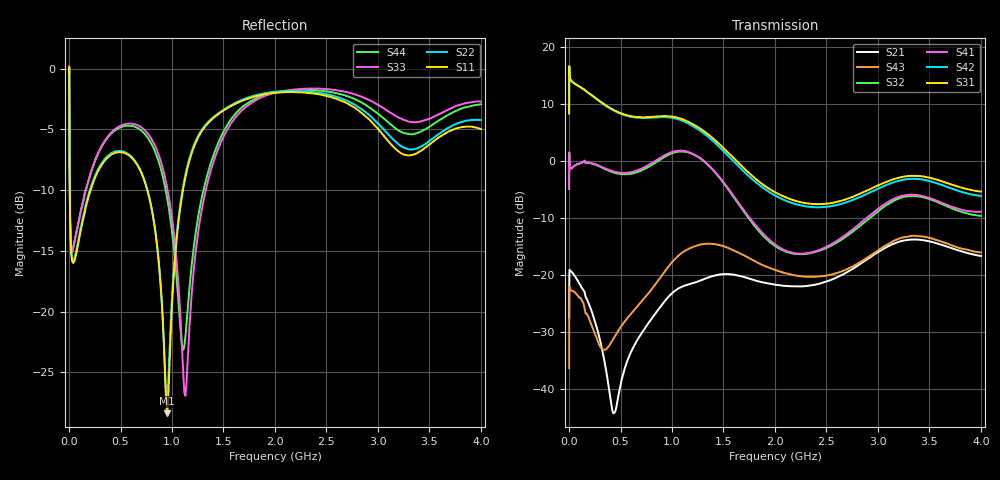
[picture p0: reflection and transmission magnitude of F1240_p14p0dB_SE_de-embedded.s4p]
! Integrated Device Technology
! Corporate Headquarters
! 6024 Silver Creek Valley Road
! San Jose, CA 95138  USA
! Phone:  1-408-284-8200
! Toll Free:  1-800-223-1366
! Webpage:  http://www.idt.com/
! Timing and RF Division
! 515 Groton Road, Suite 102
! Westford, MA 01886-6024
! Device:  F1240
! Description: Dual Intermediate Frequency Digital Variable Gain Amplifier
! Frequency:  10.0 -  500.00 MHz
! Package:  5x5 mm QFN Plastic Package: 32 pin
! Ports:  8 RF, 20 DC
!  Pin  1  = GA3 / Data  Pin 17  = RF OUT_B+
!  Pin  2  = GA4 / CLK  Pin 18  = RF OUT_B-
!  Pin  3  = GA5  Pin 19  = STBY_B
!  Pin  4  = VMODE  Pin 20  = Ground
!  Pin  5  = No Connect  Pin 21  = Ground
!  Pin  6  = GB5  Pin 22  = STB_A
!  Pin  7  = GB4  Pin 23  = RF OUT_A-  = Port 4
!  Pin  8  = GB3  Pin 24  = RF OUT_A+  = Port 3
!  Pin  9  = GB2  Pin 25  = GA0
!  Pin 10  = GB1  Pin 26  = ISET_A
!  Pin 11  = RF IN_B+  Pin 27  = VCC
!  Pin 12  = RF IN_B-  Pin 28  = Ground
!  Pin 13  = Ground  Pin 29  = RF IN_A-  = Port 2
!  Pin 14  = VCC  Pin 30  = RF IN_A+  = Port 1
!  Pin 15  = ISET_B  Pin 31  = GA1
!  Pin 16  = GB0  Pin 32  = GA2 / CSb
! Gain  = +19.5 dB
! State  = 1
! Voltage  = +5.00 V
! Current  = 85.292 mA (one channel only)
! Temperture  =  +25 C
! Test Date  =  2017-10-18
! Board  =  EB4031
! Data:  The device was measured on a custom evaluation board which has
!  individual transmission lines to the RF pins.  Data was collected
!  using a calibrated network analyzer.  The evaluation board was
!  de-embedded using Automatic Fixture Removal.
!  The reference plane is the edge of the package pin.
!  Only Channel A was measured.
!  This data is in single-ended operation.  If your needs are balanced
!  or differential S-parameters then this file needs to be used a
!  linear simulator.
! File Date:  2017-11-10  MJV
! Note:
!  Integrated Device Technology supplies this data as a sample of measured
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# Hz S dB R 100
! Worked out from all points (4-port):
!   410 points, 500 kHz to 4 GHz, reference 100 ohm
!   strongest paths, dB at 500 kHz, 930 MHz, 1.96 GHz, 2.98 GHz, 4 GHz:
!     S31: 8.3, 7.8, -5.1, -4.5, -5.4
!     S42: 8.3, 7.6, -5.7, -5.1, -6.2
!     S41: -4.9, 1.0, -14.1, -8.8, -8.9
!     S32: -4.9, 0.7, -14.4, -9.2, -9.7
!     S43: -36.4, -19.4, -18.9, -16.0, -16.1
!     S21: -27.6, -24.6, -21.6, -16.3, -16.7
!   lowest |S11| = -28.4 dB at 950 MHz (marker M1), VSWR 1.08, Z = 106 + j4.75 ohm
!   |S11| at or under -10 dB: 7.248 MHz to 209.1 MHz (201.8 MHz wide, 187 % of centre); 760 MHz to 1.106 GHz (346.3 MHz wide, 37.1 % of centre)
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500000  -0.36 -6.0  -27.51 1.7  -27.33 77.4  -60.34 65.6
        -27.56 1.6  -0.36 -5.9  -59.83 65.8  -27.32 78.5
        8.30 -105.2  -4.92 71.6  -0.45 1.2  -36.47 -144.1
        -4.94 72.7  8.28 -104.1  -36.40 -144.0  -0.46 3.5
3000000  -4.22 -55.1  -19.61 15.5  -18.41 16.1  -41.49 60.4
         -19.61 15.5  -4.19 -55.1  -41.45 60.4  -18.41 16.3
         16.00 -173.1  0.06 -5.6  -3.80 -50.6  -22.11 42.3
         0.07 -5.5  16.00 -172.9  -22.08 42.2  -3.86 -50.4
2e8  -10.25 -117.8  -25.38 -98.4  -21.09 -51.8  -34.09 10.8
     -25.47 -97.0  -10.05 -119.4  -34.06 11.1  -21.12 -51.9
     11.75 109.3  -0.43 -49.7  -8.91 -82.3  -27.28 -115.4
     -0.36 -49.8  11.71 108.6  -27.95 -113.5  -8.90 -81.6
5.4e8  -6.96 -174.7  -36.89 29.4  -22.83 -108.6  -28.06 -58.2
       -36.46 19.2  -6.87 -176.0  -28.21 -56.7  -22.98 -108.9
       8.07 24.8  -2.39 -123.1  -4.58 -152.0  -29.44 48.5
       -2.15 -124.3  7.97 23.8  -28.20 33.8  -4.73 -151.9
9.5e8  -28.37 35.8  -23.12 -60.9  -20.32 167.6  -23.63 -154.8
       -24.18 -70.5  -27.51 28.3  -23.96 -149.8  -20.73 167.0
       7.80 -75.0  0.87 146.5  -9.68 143.3  -19.78 -43.9
       1.14 142.0  7.61 -76.8  -18.92 -58.7  -10.53 146.3
1.52e9  -3.34 -146.9  -19.56 153.3  -26.17 34.3  -25.72 70.4
        -19.88 157.6  -3.28 -147.1  -25.59 76.2  -27.36 33.2
        1.86 123.9  -4.39 -37.7  -5.28 -130.5  -15.36 144.8
        -4.24 -42.8  1.33 122.6  -15.12 139.2  -4.89 -133.9
4e9  -4.98 -155.8  -16.75 63.0  -21.44 -46.5  -19.82 -48.3
     -16.72 62.3  -4.24 -150.3  -22.11 -29.5  -24.77 -34.6
     -5.41 10.1  -9.67 -117.1  -2.72 -136.9  -15.50 90.8
     -8.95 -128.4  -6.17 19.3  -16.09 63.4  -2.94 -142.5
